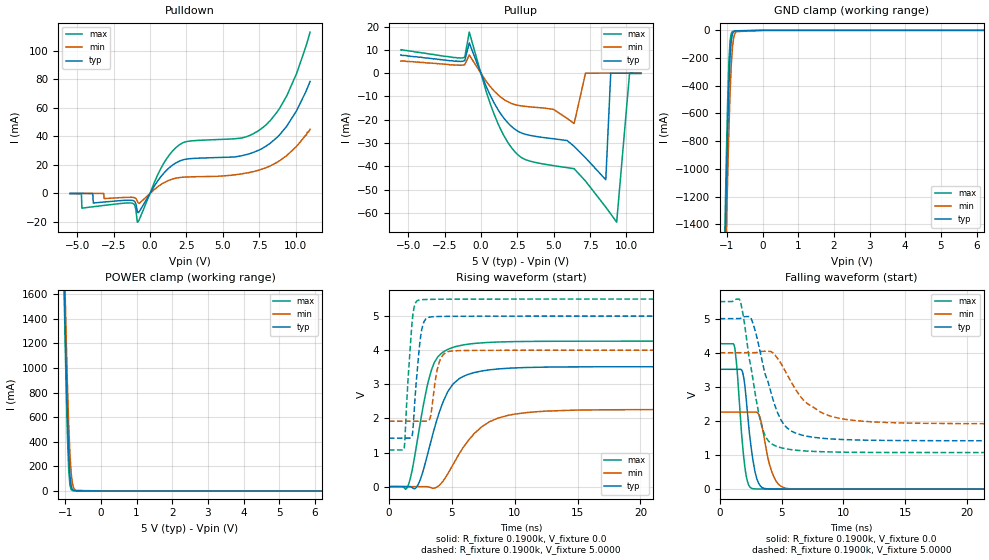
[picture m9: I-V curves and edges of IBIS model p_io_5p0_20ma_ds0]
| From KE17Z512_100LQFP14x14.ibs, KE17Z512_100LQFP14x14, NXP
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[Model] p_io_5p0_20ma_ds0
|   Model p_io_5p0_20ma_ds0
| This model was characterised for following simulation conditions:
| External (pad) voltage:
|   - Typ: 5.0V,   - Min: 4.0V,   - Max: 5.5V
| Library cells for typ/min/max conditions are connected as defined below:
|  pad - External Pad
|  ipp_do_lv - Core Input
|  ipp_obe_lv - Output Buffer Enable
|  abt_close_nor_rst_mv - vdde
|  dvdd - dvdd
|  dvss - dvss
|  esd_boost - vdde
|  ipp_dse_lv - dvss
|  ipp_ina_280_mv - NC
|  ipp_ina_40_a_mv - NC
|  ipp_ina_40_b_mv - NC
|  ipp_ina_40_c_mv - NC
|  ipp_ina_40_d_mv - NC
|  ipp_ina_40_e_mv - NC
|  ipp_ina_40_f_mv - NC
|  ipp_ina_40_g_mv - NC
|  ipp_ina_40_h_mv - NC
|  ipp_ind_lv - NC
|  vdde - vdde
|  vsse - vsse
| All other pins connected to ground
Model_type I/O
Polarity   Non-Inverting
Enable   Active-High
Vinl =   1.5000V
Vinh =   3.5000V
Vmeas =  2.5000V
Cref =   50.0000F
C_comp   2.8015pF   2.6791pF   2.9922pF
[Model Spec]
| variable   typ   min   max
Vinh   3.5000V   2.8000V   3.8500V
Vinl   1.5000V   1.2000V   1.6500V
S_overshoot_high   5.3000V   4.3000V   5.8000V
S_overshoot_low   -0.3000V   -0.3000V   -0.3000V
Vmeas   2.5000V   2.0000V   2.7500V
[Temperature Range]   25.0000   0.1250k   -40.0000
[Voltage Range]   5.0000V   4.0000V   5.5000V
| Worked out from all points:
|   slope of the pulldown table from 0 to 0.75 V, typ, clamps not added: 63.4 ohm
|   slope of the pullup table from 0 to 0.75 V, typ, clamps not added: 69.3 ohm
|   rising waveform, R_fixture 0.1900k, V_fixture 0.0: 20-80 % time 1.83ns typ, 2.8ns min, 1.34ns max; typ from 0 V to 3.52 V
|   rising waveform, R_fixture 0.1900k, V_fixture 5.0000: 20-80 % time 487ps typ, 526ps min, 450ps max; typ from 1.42 V to 5 V
|   falling waveform, R_fixture 0.1900k, V_fixture 0.0: 20-80 % time 653ps typ, 824ps min, 541ps max; typ from 3.52 V to 0 V
|   falling waveform, R_fixture 0.1900k, V_fixture 5.0000: 20-80 % time 1.69ns typ, 2.72ns min, 1.22ns max; typ from 5 V to 1.42 V
[Pulldown]
|Voltage   I(typ)   I(min)   I(max)
-5.5V     -20uA      0A         -140uA
-4.718V   -10uA      10uA       -260uA
-4.684V   -10uA      10uA       -10.32mA
-3.902V   -6.7mA     10uA       -9.32mA
-1.216V   -4.868mA   -2.733mA   -6.875mA
-842mV    -13.35mA   -6.039mA   -20.16mA
722mV     11.49mA    6.076mA    17.11mA
1.98V     22.45mA    11.06mA    33.79mA
6.604V    27.2mA     14.3mA     39.67mA
8.236V    35mA       19.2mA     50.7mA
9.392V    47.1mA     26.5mA     68.3mA
11V       78.5mA     45mA       113.1mA
[Pullup]
|Voltage   I(typ)   I(min)   I(max)
-5.5V     7.8mA      5.2mA      10mA
-1.206V   5.17mA     3.47mA     6.63mA
-798mV    12.96mA    7.798mA    17.62mA
902mV     -12.68mA   -7.61mA    -17.51mA
2.194V    -23.35mA   -13.2mA    -32.67mA
6.41V     -31.44mA   -21.63mA   -40.99mA
7.192V    -36.3mA    -10uA      -46.3mA
8.586V    -45.74mA   10uA       -57.49mA
8.926V    -50uA      0A         -60.38mA
9.334V    -10uA      0A         -63.94mA
10.22V    -10uA      -10uA      -190uA
11V       -30uA      0A         -140uA
[GND_clamp]
|Voltage   I(typ)   I(min)   I(max)
-5.5V     -74.62A    -74.49A    -74.76A
-1.08V    -1.983A    -2.319A    -1.787A
-1.046V   -1.53A     -1.877A    -1.323A
-1.012V   -1.108A    -1.459A    -893.4mA
-978mV    -729.3mA   -1.075A    -519.1mA
-944mV    -416.7mA   -736.6mA   -235.7mA
-910mV    -195.2mA   -457.3mA   -77.19mA
-876mV    -73.87mA   -251.2mA   -21.92mA
-842mV    -25.05mA   -121.5mA   -8.825mA
-740mV    -3.106mA   -9.724mA   -4.306mA
0V        -97.39pA   -840.9pA   -997.7pA
11V       0A         0A         0A
[POWER_clamp]
|Voltage   I(typ)   I(min)   I(max)
-5.5V     79A        78.7A      79.25A
-1.036V   1.833A     2.072A     1.706A
-1.002V   1.371A     1.626A     1.227A
-968mV    946.6mA    1.212A     789.9mA
-934mV    579.8mA    842.9mA    422.7mA
-900mV    297mA      533.2mA    167mA
-866mV    120.4mA    298.4mA    45.78mA
-832mV    39.59mA    145.6mA    10.75mA
-798mV    11.97mA    63.04mA    3.299mA
-696mV    1.006mA    4.196mA    1.128mA
0V        141.3pA    3.127nA    117.5pA
11V       0A         0A         0A
[Ramp]
| variable   typ   min   max
dV/dt_r  2.1092/1.8313n   1.3560/2.8020n   2.5591/1.3390n
dV/dt_f  2.1481/1.6950n   1.2495/2.7214n   2.6559/1.2223n
R_load = 0.1900k
[Rising Waveform]
R_fixture= 0.1900k
V_fixture= 0.0
V_fixture_min= 0.0
V_fixture_max= 0.0
|time   V(typ)   V(min)   V(max)
0s        3.915nV    44.52nV    29.77nV
1.422ns   105.6uV    -3.51uV    -47.3mV
2.222ns   -4.543mV   48.03uV    1.26V
2.968ns   791.1mV    233.8uV    2.809V
3.62ns    1.708V     -44.24mV   3.643V
4.303ns   2.479V     158.6mV    3.942V
5.316ns   3.078V     789.3mV    4.108V
7.382ns   3.39V      1.755V     4.216V
10.69ns   3.491V     2.161V     4.257V
40ns      3.515V     2.26V      4.265V
[Rising Waveform]
R_fixture= 0.1900k
V_fixture= 5.0000
V_fixture_min= 4.0000
V_fixture_max= 5.5000
|time   V(typ)   V(min)   V(max)
0s        1.42V      1.917V     1.073V
1.213ns   1.42V      1.918V     1.126V
1.875ns   1.545V     1.918V     4.93V
2.342ns   3.765V     1.918V     5.466V
2.621ns   4.616V     1.918V     5.482V
2.922ns   4.912V     1.918V     5.488V
3.33ns    4.976V     2.088V     5.491V
4.051ns   4.99V      3.695V     5.495V
4.973ns   4.995V     3.975V     5.497V
40ns      5V         4V         5.5V
[Falling Waveform]
R_fixture= 0.1900k
V_fixture= 0.0
V_fixture_min= 0.0
V_fixture_max= 0.0
|time   V(typ)   V(min)   V(max)
0s        3.515V     2.26V      4.265V
1.203ns   3.515V     2.26V      4.165V
1.41ns    3.515V     2.26V      3.488V
1.914ns   3.325V     2.26V      1.026V
2.213ns   2.361V     2.26V      260.4mV
2.573ns   1.131V     2.26V      25.7mV
3.3ns     84.47mV    2.049V     4.224mV
4.237ns   5.122mV    480.2mV    2.023mV
5.351ns   2.175mV    26.66mV    985.2uV
40ns      154.1nV    422.6nV    104.3nV
[Falling Waveform]
R_fixture= 0.1900k
V_fixture= 5.0000
V_fixture_min= 4.0000
V_fixture_max= 5.5000
|time   V(typ)   V(min)   V(max)
0s        5V         4V         5.5V
1.611ns   5.002V     4V         5.555V
1.892ns   5.047V     4V         5.114V
2.487ns   5.037V     4V         3.656V
3.072ns   4.35V      4.014V     2.375V
3.576ns   3.517V     4.044V     1.643V
4.821ns   2.127V     3.761V     1.228V
6.809ns   1.571V     2.593V     1.122V
10.07ns   1.454V     2.052V     1.084V
40ns      1.42V      1.918V     1.073V
